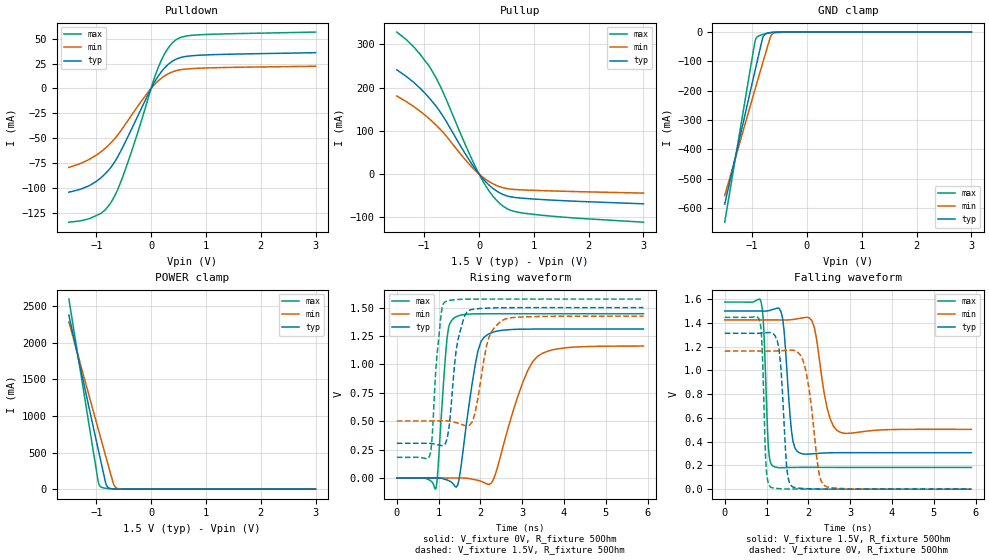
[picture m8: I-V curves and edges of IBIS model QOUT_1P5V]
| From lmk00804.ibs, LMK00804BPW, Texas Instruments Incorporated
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|   Model QOUT 1.5VCC
[Model]   QOUT_1P5V
Model_type   3-state
Polarity   Non-Inverting
Vmeas = 0.75
Vref = 1.5
Cref = 15pF
Rref = 50
|   typ   min   max
|   (fast PVT)   (slow PVT)   (nom PVT)
C_comp   0.315p   0.300p   0.317p
|C_comp (Hi state)   0.315p   0.300p   0.317p
|C_comp (Low state)   0.358p   0.325p   0.360p
[Voltage Range]   1.5   1.425   1.575
[Temperature Range]   45   125   -40
[Pullup Reference]   1.5   1.425   1.575
[Pulldown Reference]   -0   0   0
[Power Clamp Reference]   1.5   1.425   1.575
[GND Clamp Reference]   0   0   0
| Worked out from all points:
|   slope of the pulldown table from 0 to 0.225 V, typ, clamps not added: 11.7 ohm
|   slope of the pullup table from 0 to 0.225 V, typ, clamps not added: 7.41 ohm
|   GND clamp passes 1 mA (typ) near -0.64 V on its own axis
|   POWER clamp passes 1 mA (typ) near -0.60 V on its own axis
|   falling waveform, V_fixture 1.5V, R_fixture 50Ohm: 20-80 % time 147ps typ, 239ps min, 88.3ps max; typ from 1.5 V to 0.307 V
|   rising waveform, V_fixture 0V, R_fixture 50Ohm: 20-80 % time 312ps typ, 603ps min, 163ps max; typ from 0 V to 1.31 V
|   rising waveform, V_fixture 1.5V, R_fixture 50Ohm: 20-80 % time 216ps typ, 273ps min, 159ps max; typ from 0.306 V to 1.5 V
|   falling waveform, V_fixture 0V, R_fixture 50Ohm: 20-80 % time 131ps typ, 237ps min, 75.9ps max; typ from 1.31 V to 0 V
[Pulldown]
|   Voltage   I(typ)   I(min)   I(max)
-1.5V     -104.4mA   -79.45mA   -134.6mA
-1.163V   -98.67mA   -72.33mA   -131.6mA
-919.5mV  -90.09mA   -63.92mA   -125.8mA
-717mV    -78.19mA   -53.81mA   -113.4mA
-541.5mV  -61.77mA   -41.77mA   -92.51mA
-375mV    -43.08mA   -28.43mA   -66.58mA
-1.5mV    -164.8uA   -99.93uA   -282.8uA
129mV     12.34mA    7.511mA    20.96mA
291mV     23.12mA    14.08mA    38.87mA
444mV     29.08mA    17.66mA    48.48mA
885mV     33.4mA     20.34mA    53.96mA
3V        35.94mA    22.32mA    56.67mA
[GND Clamp]
|   Voltage   I(typ)   I(min)   I(max)
-1.5V     -586.6mA   -557.7mA   -648.1mA
-955.5mV  -138.9mA   -201mA     -39.92mA
-937.5mV  -124.2mA   -189.4mA   -25.42mA
-910.5mV  -102.3mA   -171.9mA   -16.8mA
-825mV    -33.15mA   -116.9mA   -9.221mA
-798mV    -15.7mA    -99.61mA   -7.705mA
-771mV    -8.258mA   -82.38mA   -6.3mA
-739.5mV  -4.588mA   -62.36mA   -4.804mA
-667.5mV  -1.615mA   -17.58mA   -2.108mA
-631.5mV  -936.2uA   -6.481mA   -1.211mA
-591mV    -464uA     -2.158mA   -566.9uA
3V        0A         0A         0A
[Pullup]
|   Voltage   I(typ)   I(min)   I(max)
-1.5V     241.2mA    180.6mA    328.7mA
-1.194V   212.5mA    156.4mA    294.8mA
-879mV    171.7mA    124.7mA    243.7mA
-672mV    136.9mA    98.65mA    194.1mA
-240mV    44.52mA    31.45mA    64.95mA
7.5mV     -1.223mA   -837.5uA   -1.845mA
210mV     -28.8mA    -19.61mA   -44.16mA
408mV     -45.75mA   -30.83mA   -71.51mA
525mV     -51.31mA   -34.27mA   -81.24mA
633mV     -54.03mA   -35.79mA   -86.42mA
948mV     -57.63mA   -37.68mA   -92.91mA
3V        -69.16mA   -44.34mA   -111.7mA
[POWER Clamp]
|   Voltage   I(typ)   I(min)   I(max)
-1.5V     2.379A     2.288A     2.598A
-969mV    558mA      833.6mA    122.5mA
-951mV    496.9mA    784.7mA    64.29mA
-919.5mV  390mA      699.2mA    29.73mA
-834mV    100.7mA    467.8mA    12.93mA
-811.5mV  49.51mA    407mA      10.88mA
-762mV    13.58mA    273.6mA    7.058mA
-685.5mV  3.765mA    71.77mA    2.905mA
-649.5mV  2.239mA    26.42mA    1.694mA
-604.5mV  1.088mA    7.883mA    763.6uA
3V        0A         0A         0A
[Ramp]
R_load = 50
|   typ   min   max
dV/dt_r   0.787188/3.12139e-10   0.697013/6.02998e-10   0.86756/1.62985e-10
dV/dt_f   0.715904/1.46835e-10   0.552705/2.3934e-10   0.835223/8.83402e-11
[Falling Waveform]
V_fixture = 1.5V
V_fixture_min = 1.425V
V_fixture_max = 1.575V
R_fixture = 50Ohm
C_fixture = 0F
|   Time   V(typ)   V(min)   V(max)
0s        1.5V       1.425V     1.575V
874.5ps   1.499V     1.425V     1.569V
1.04ns    1.502V     1.425V     385mV
1.163ns   1.514V     1.425V     193.2mV
1.384ns   1.438V     1.424V     181mV
1.595ns   497.6mV    1.427V     183mV
1.764ns   310.5mV    1.436V     183.6mV
2.147ns   299.4mV    1.359V     183.7mV
2.688ns   307.2mV    493.4mV    183.4mV
5.9ns     306.8mV    503.8mV    183mV
[Rising Waveform]
V_fixture = 0V
V_fixture_min = 0V
V_fixture_max = 0V
R_fixture = 50Ohm
C_fixture = 0F
|   Time   V(typ)   V(min)   V(max)
0s        485.1pV    18.82nV    400.4pV
938.7ps   1.186mV    727.8uV    -88.02mV
1.201ns   -16.03mV   931.1uV    1.229V
1.389ns   -70.73mV   1.077mV    1.413V
1.508ns   29.15mV    1.169mV    1.431V
1.879ns   1.004V     -14.91mV   1.445V
2.085ns   1.237V     -38.63mV   1.445V
2.302ns   1.284V     -19.62mV   1.446V
3.367ns   1.311V     1.071V     1.446V
5.9ns     1.312V     1.162V     1.446V
[Rising Waveform]
V_fixture = 1.5V
V_fixture_min = 1.425V
V_fixture_max = 1.575V
R_fixture = 50Ohm
C_fixture = 0F
|   Time   V(typ)   V(min)   V(max)
0s        306.1mV    502.5mV    182.6mV
786ps     306.4mV    502.6mV    195.7mV
1.04ns    288.1mV    503.6mV    1.369V
1.163ns   305mV      503.8mV    1.552V
1.454ns   1.198V     483.9mV    1.571V
1.725ns   1.474V     460mV      1.574V
1.869ns   1.487V     568.1mV    1.574V
2.207ns   1.496V     1.243V     1.575V
2.517ns   1.498V     1.386V     1.575V
5.9ns     1.5V       1.425V     1.575V
[Falling Waveform]
|Gnd
V_fixture = 0V
V_fixture_min = 0V
V_fixture_max = 0V
R_fixture = 50Ohm
C_fixture = 0F
|   Time   V(typ)   V(min)   V(max)
0s        1.312V     1.163V     1.446V
849.2ps   1.313V     1.163V     1.404V
992.5ps   1.317V     1.162V     173.5mV
1.097ns   1.318V     1.162V     17.92mV
1.301ns   1.177V     1.165V     4.577mV
1.483ns   180.7mV    1.169V     2.029mV
1.595ns   27.83mV    1.17V      1.4mV
1.943ns   4.742mV    996.1mV    1.066mV
2.393ns   1.602mV    28.59mV    724.7uV
5.9ns     374.5uV    548.7uV    249.6uV
